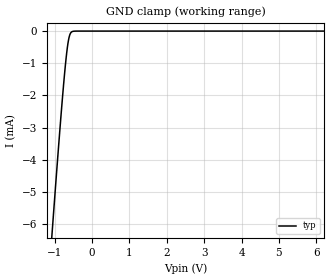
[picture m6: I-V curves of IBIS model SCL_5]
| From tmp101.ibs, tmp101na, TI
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|   SCL 5 V Model
[Model]   SCL_5
Model_type   Input
Vinl = 1.5
Vinh = 3.5
|   typ   min   max
C_comp   4.014pF   NA   NA
[Voltage Range]   5   NA   NA
[Temperature Range]   27   NA   NA
[Power Clamp Reference]   5   NA   NA
[GND Clamp Reference]   0   NA   NA
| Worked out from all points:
|   GND clamp passes 1 mA (typ) near -0.71 V on its own axis
[GND Clamp]
|   Voltage   I(typ)   I(min)   I(max)
-5V       -71.88mA   NA         NA
-1.129V   -7.217mA   NA         NA
-1.043V   -5.854mA   NA         NA
-914.4mV  -3.868mA   NA         NA
-827mV    -2.572mA   NA         NA
-740.2mV  -1.389mA   NA         NA
-680.4mV  -698.3uA   NA         NA
-646.1mV  -392uA     NA         NA
-616.7mV  -204.8uA   NA         NA
-581.6mV  -77.75uA   NA         NA
-518.8mV  -10.71uA   NA         NA
9.985V    0A         NA         NA
[POWER Clamp]
|   SCR cell for ESD function. Effects occurr above VDD x 2
|   Voltage   I(typ)   I(min)   I(max)
-5V       0A         NA         NA
0V        0A         NA         NA
10V       0A         NA         NA
